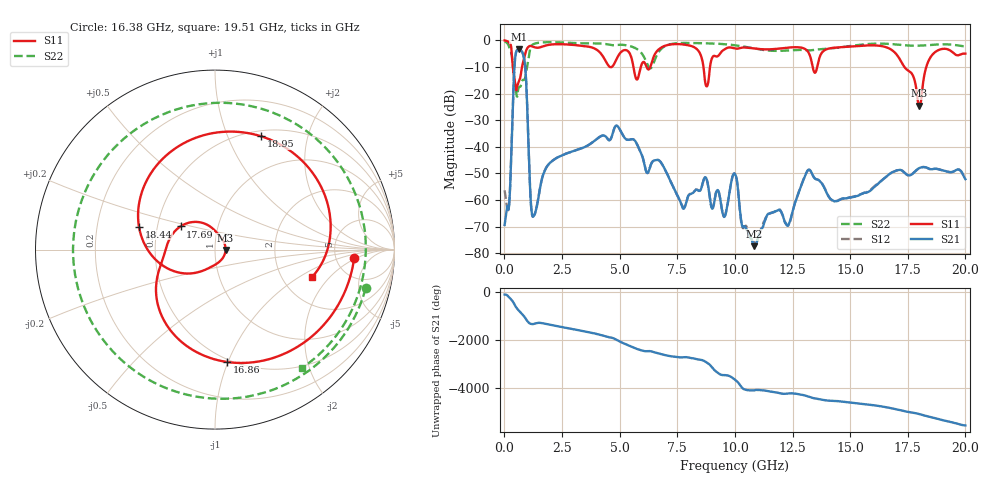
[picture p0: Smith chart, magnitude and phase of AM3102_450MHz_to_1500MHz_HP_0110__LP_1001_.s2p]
!Agilent Technologies,E8364B,MY43040894,A.07.50.67
!Agilent E8364B: A.07.50.67
!Date: Thursday, January 11, 2018 05:48:22
!Correction: S11(Full 2 Port(1,2))
!S21(Full 2 Port(1,2))
!S12(Full 2 Port(1,2))
!S22(Full 2 Port(1,2))
!S2P File: Measurements: S11, S21, S12, S22:
# Hz S  dB  R 50
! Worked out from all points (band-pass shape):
!   1601 points, 10 MHz to 20 GHz, reference 50 ohm
!   highest |S21| = -3.36 dB at 622.2 MHz (marker M1); lowest = -77.3 dB at 10.84 GHz (marker M2)
!   |S21| within 3 dB of the highest: 471.6 MHz to 843.7 MHz (372.2 MHz wide, 56.6 % of centre)
!   lowest |S11| = -24.6 dB at 18 GHz (marker M3), VSWR 1.13, Z = 56.3 - j0.234 ohm
!   |S11| at or under -10 dB: 369.2 MHz to 765.8 MHz (396.6 MHz wide, 69.9 % of centre); 5.599 GHz to 5.919 GHz (319.7 MHz wide, 5.55 % of centre); 17.35 GHz to 18.3 GHz (951 MHz wide, 5.33 % of centre)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
!   |S22| runs from -21.1 to -0.5 dB; largest |S21 - S12| = 0.0029
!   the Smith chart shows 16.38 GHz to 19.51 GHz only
!   S11 on the Smith chart (normalised r, x): 16.38 GHz: 7.51, -1.82; 16.86 GHz: 0.48, -0.99; 17.69 GHz: 0.66, +0.18; 18.44 GHz: 0.39, +0.13; 18.95 GHz: 0.56, +1.33; 19.51 GHz: 2.91, -1.31
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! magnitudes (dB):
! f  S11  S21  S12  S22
! 10 MHz  -0.1  -69.3  -56.3  -0.5
! 197.4 MHz  -0.7  -62.5  -62.7  -2.3
! 447.3 MHz  -15.2  -8.7  -8.7  -15.3
! 622.2 MHz  -15.6  -3.4  -3.4  -17.7
! 884.6 MHz  -5.8  -8.4  -8.5  -14.6
! 1.259 GHz  -2.5  -66.0  -66.1  -1.5
! 3.346 GHz  -2.0  -40.5  -40.6  -1.1
! 6.682 GHz  -3.5  -45.0  -44.9  -4.6
! 7.769 GHz  -1.6  -63.2  -62.8  -1.0
! 8.781 GHz  -17.3  -52.3  -52.3  -1.1
! 10.01 GHz  -3.1  -50.2  -50.0  -1.9
! 10.84 GHz  -3.1  -77.3  -76.1  -3.1
! 13.34 GHz  -8.6  -50.0  -50.0  -3.7
! 16.38 GHz  -2.2  -52.6  -52.6  -1.2
! 16.68 GHz  -3.0  -50.4  -50.4  -1.4
! 16.86 GHz  -4.0  -49.4  -49.4  -1.5
! 17.69 GHz  -12.7  -50.3  -50.2  -2.0
! 18 GHz  -24.6  -47.9  -48.0  -2.0
! 18.44 GHz  -7.1  -48.3  -48.4  -1.8
! 18.95 GHz  -3.3  -48.7  -48.7  -1.5
! 19.51 GHz  -5.0  -49.2  -49.1  -1.7
! 20 GHz  -5.0  -52.1  -52.0  -2.3
